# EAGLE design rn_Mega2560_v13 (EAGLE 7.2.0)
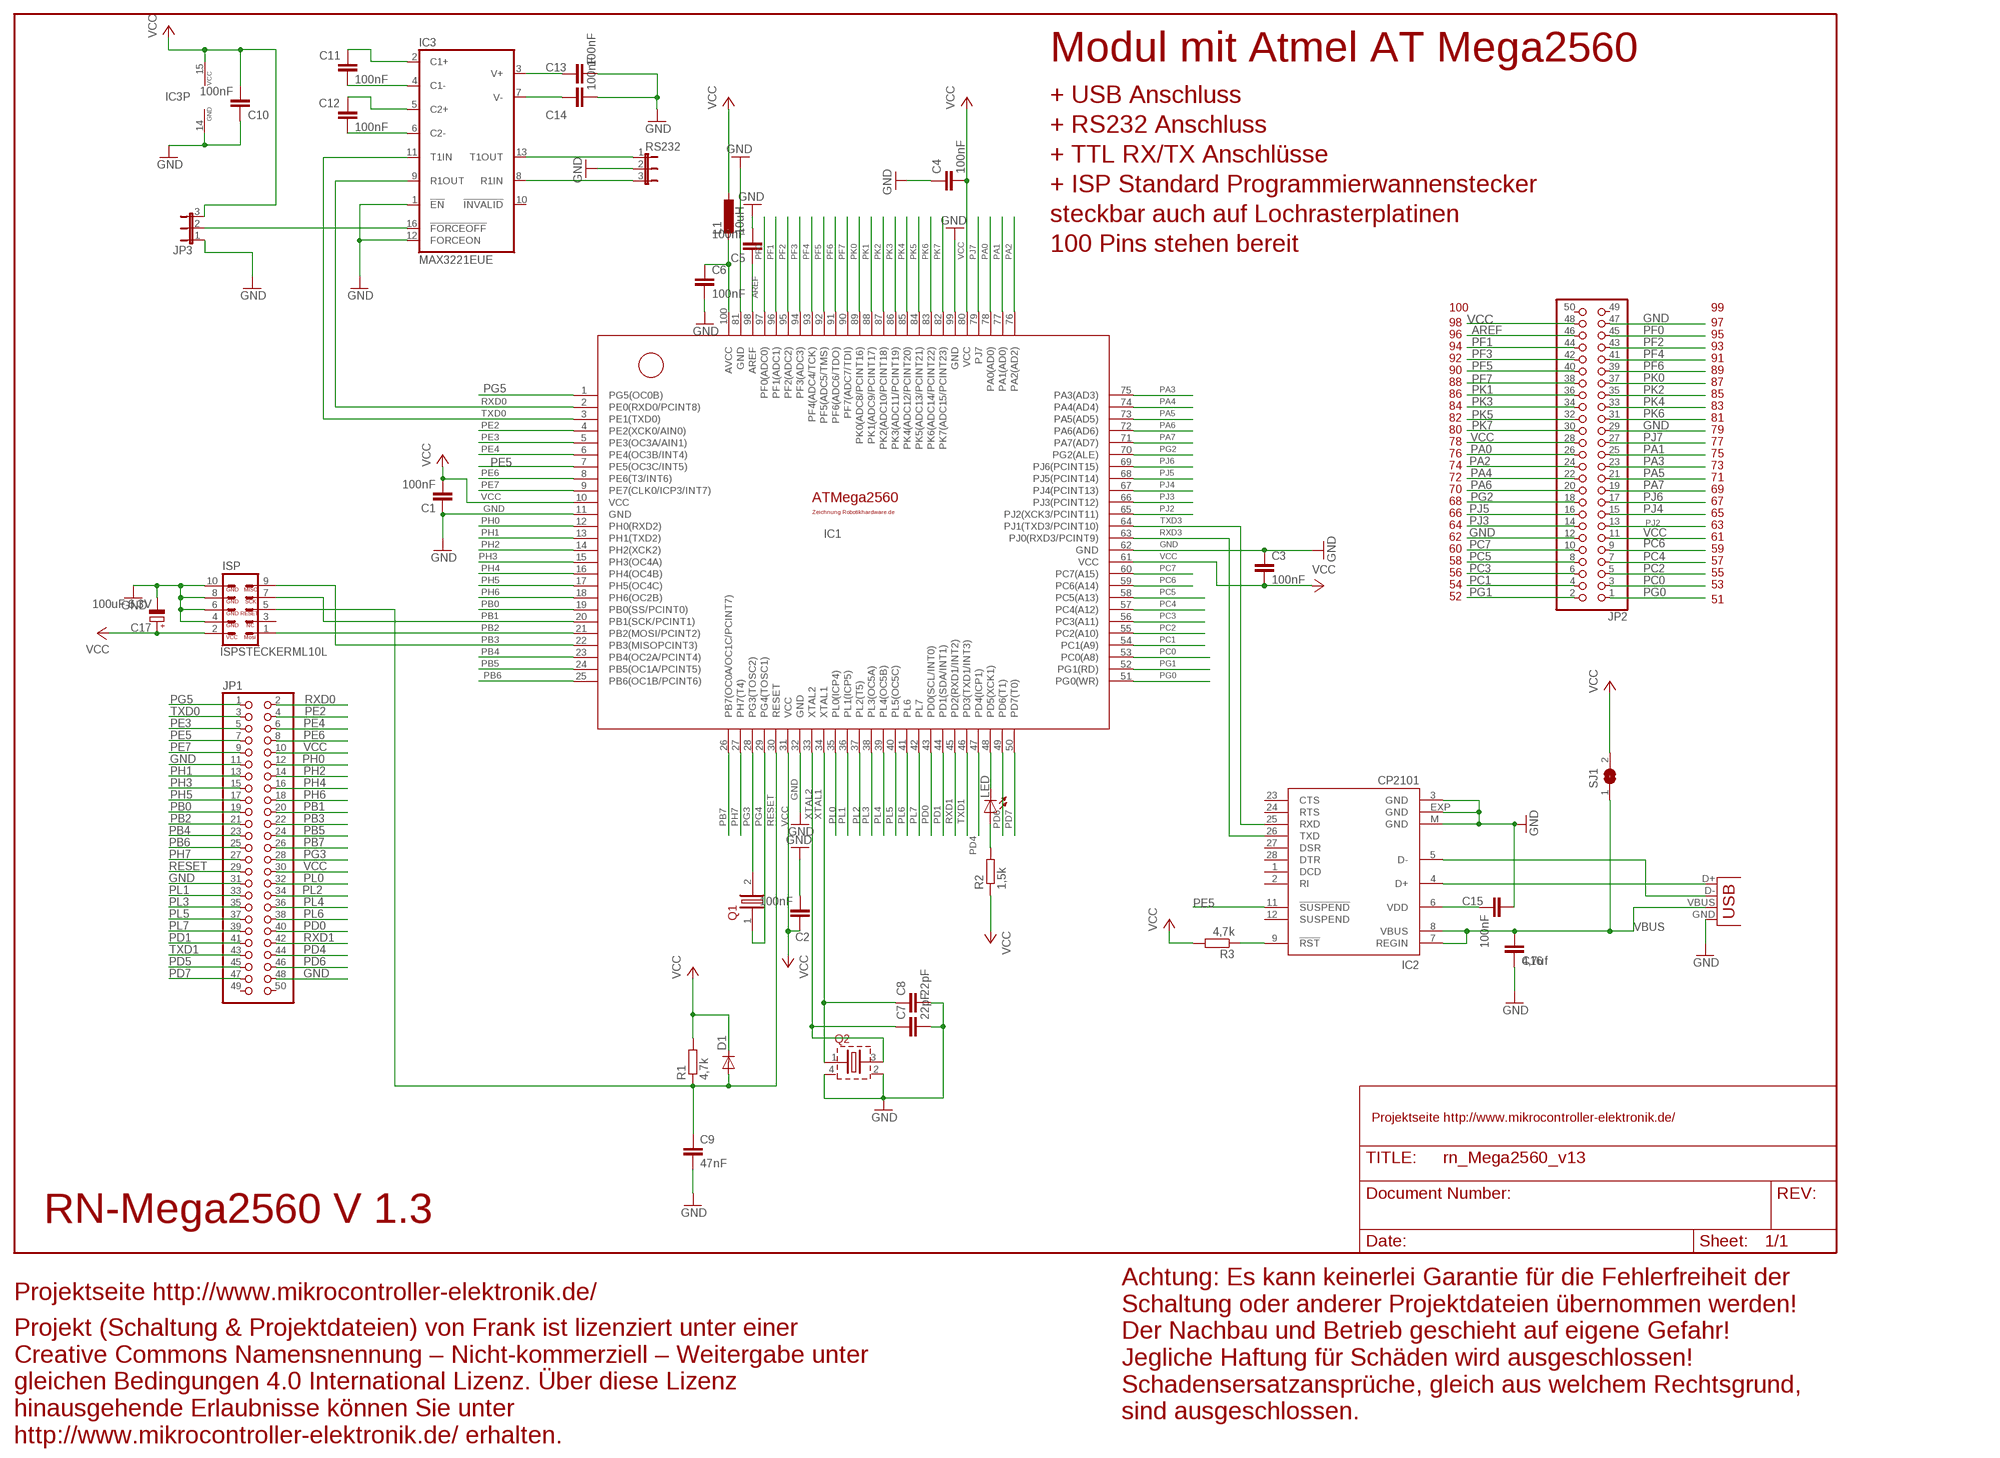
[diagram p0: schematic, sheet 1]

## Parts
C1  100nF  C-EUC0603  [C0603]
C2  100nF  C-EUC0603  [C0603]
C3  100nF  C-EUC0603  [C0603]
C4  100nF  C-EUC0603  [C0603]
C5  100nF  C-EUC0603  [C0603]
C6  100nF  C-EUC0603  [C0603]
C7  22pF  C-EUC0603  [C0603]
C8  22pF  C-EUC0603  [C0603]
C9  47nF  C-EUC0603  [C0603]
C10  100nF  C-EUC0603  [C0603]
C11  100nF  C-EUC0603  [C0603]
C12  100nF  C-EUC0603  [C0603]
C13  100nF  C-EUC0603  [C0603]
C14  100nF  C-EUC0603  [C0603]
C15  100nF  C-EUC0603  [C0603]
C16  4,7uf  C-EUC1206  [C1206]
C17  100uF 6,3V  CPOL-EU085CS-1AR  [085CS_1AR]
D1  DIODE-MINIMELF  [MINIMELF]
IC1  ATMEGA2560PINGLEICH  [TQFP100]
IC2  CP2101  [MLP28]
IC3  MAX3221EUE  [TSSOP16]
ISP  ISPSTECKERML10L  [ML10L]
JP1  PINHD-2X25  [2X25]
JP2  PINHD-2X25  [2X25]
JP3  JP2W  [JP2W]
L1  10uH  L-EUL3225M  [L3225M]
LED  LEDCHIPLED_0805  [CHIPLED_0805]
Q1  FC135QUARZ  [FC135QUARZ]
Q2  KS7QUARZ  [KX7QUARZ]
R1  4,7k  R-EU_M0805  [M0805]
R2  1,5k  R-EU_M0805  [M0805]
R3  4,7k  R-EU_M0805  [M0805]
RS232  JP2W  [JP2W]
SJ1  SJW  [SJW]
USB  USB-MB-H  [USB-MB-H]

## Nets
AREF: C5.1 IC1.98(AREF) JP2.46
AVCC: C6.1 IC1.100(AVCC) L1.2
GND: C1.1 C2.2 C3.1 C4.1 C5.2 C6.2 C7.2 C8.2 C9.2 C10.1 C13.2 C14.2 C15.1 C16.2 C17.- IC1.11(GND) IC1.32(GND) IC1.62(GND) IC1.81(GND) IC1.99(GND) IC2.3(GND) IC2.EXP(GND) IC2.M(GND) IC3.1(!EN) IC3.12(FORCEON) IC3.14(GND) ISP.4 ISP.6 ISP.8 ISP.10 JP1.11 JP1.31 JP1.48 JP2.12 JP2.29 JP2.47 JP3.1 Q2.2(GND) Q2.4(GND) RS232.2 USB.GND
N$9: C12.2 IC3.6(C2-)
N$10: C12.1 IC3.5(C2+)
N$11: C11.2 IC3.4(C1-)
N$12: IC2.5(D-) USB.D-
N$15: C11.1 IC3.2(C1+)
N$16: LED.A R2.2
N$18: IC2.9(!RST) R3.1
N$21: IC3.8(R1IN) RS232.3
N$22: C13.1 IC3.3(V+)
N$23: C14.1 IC3.7(V-)
N$24: IC3.16(!FORCEOFF) JP3.2
N$28: IC2.4(D+) USB.D+
N$29: C15.2 IC2.6(VDD)
PA0: IC1.78(PA0(AD0)) JP2.26
PA1: IC1.77(PA1(AD0)) JP2.25
PA2: IC1.76(PA2(AD2)) JP2.24
PA3: IC1.75(PA3(AD3)) JP2.23
PA4: IC1.74(PA4(AD4)) JP2.22
PA5: IC1.73(PA5(AD5)) JP2.21
PA6: IC1.72(PA6(AD6)) JP2.20
PA7: IC1.71(PA7(AD7)) JP2.19
PB0: IC1.19(PB0(SS/PCINT0)) JP1.19
PB1: IC1.20(PB1(SCK/PCINT1)) ISP.7 JP1.20
PB2: IC1.21(PB2(MOSI/PCINT2)) ISP.1 JP1.21
PB3: IC1.22(PB3(MISOPCINT3)) ISP.9 JP1.22
PB4: IC1.23(PB4(OC2A/PCINT4)) JP1.23
PB5: IC1.24(PB5(OC1A/PCINT5)) JP1.24
PB6: IC1.25(PB6(OC1B/PCINT6)) JP1.25
PB7: IC1.26(PB7(OC0A/OC1C/PCINT7)) JP1.26
PC0: IC1.53(PC0(A8)) JP2.3
PC1: IC1.54(PC1(A9)) JP2.4
PC2: IC1.55(PC2(A10)) JP2.5
PC3: IC1.56(PC3(A11)) JP2.6
PC4: IC1.57(PC4(A12)) JP2.7
PC5: IC1.58(PC5(A13)) JP2.8
PC6: IC1.59(PC6(A14)) JP2.9
PC7: IC1.60(PC7(A15)) JP2.10
PD0: IC1.43(PD0(SCL/INT0)) JP1.40
PD1: IC1.44(PD1(SDA/INT1)) JP1.41
PD4: IC1.47(PD4(ICP1)) JP1.44
PD5: IC1.48(PD5(XCK1)) JP1.45 LED.C
PD6: IC1.49(PD6(T1)) JP1.46
PD7: IC1.50(PD7(T0)) JP1.47
PE2: IC1.4(PE2(XCK0/AIN0)) JP1.4
PE3: IC1.5(PE3(OC3A/AIN1)) JP1.5
PE4: IC1.6(PE4(OC3B/INT4)) JP1.6
PE5: IC1.7(PE5(OC3C/INT5)) IC2.11(!SUSPEND) JP1.7
PE6: IC1.8(PE6(T3/INT6)) JP1.8
PE7: IC1.9(PE7(CLK0/ICP3/INT7)) JP1.9
PF0: IC1.97(PF0(ADC0)) JP2.45
PF1: IC1.96(PF1(ADC1)) JP2.44
PF2: IC1.95(PF2(ADC2)) JP2.43
PF3: IC1.94(PF3(ADC3)) JP2.42
PF4: IC1.93(PF4(ADC4/TCK)) JP2.41
PF5: IC1.92(PF5(ADC5/TMS)) JP2.40
PF6: IC1.91(PF6(ADC6/TDO)) JP2.39
PF7: IC1.90(PF7(ADC7/TDI)) JP2.38
PG0: IC1.51(PG0(WR)) JP2.1
PG1: IC1.52(PG1(RD)) JP2.2
PG2: IC1.70(PG2(ALE)) JP2.18
PG3: IC1.28(PG3(TOSC2)) JP1.28 Q1.2
PG4: IC1.29(PG4(TOSC1)) Q1.1
PG5: IC1.1(PG5(OC0B)) JP1.1
PH0: IC1.12(PH0(RXD2)) JP1.12
PH1: IC1.13(PH1(TXD2)) JP1.13
PH2: IC1.14(PH2(XCK2)) JP1.14
PH3: IC1.15(PH3(OC4A)) JP1.15
PH4: IC1.16(PH4(OC4B)) JP1.16
PH5: IC1.17(PH5(OC4C)) JP1.17
PH6: IC1.18(PH6(OC2B)) JP1.18
PH7: IC1.27(PH7(T4)) JP1.27
PJ2: IC1.65(PJ2(XCK3/PCINT11)) JP2.13
PJ3: IC1.66(PJ3(PCINT12)) JP2.14
PJ4: IC1.67(PJ4(PCINT13)) JP2.15
PJ5: IC1.68(PJ5(PCINT14)) JP2.16
PJ6: IC1.69(PJ6(PCINT15)) JP2.17
PJ7: IC1.79(PJ7) JP2.27
PK0: IC1.89(PK0(ADC8/PCINT16)) JP2.37
PK1: IC1.88(PK1(ADC9/PCINT17)) JP2.36
PK2: IC1.87(PK2(ADC10/PCINT18)) JP2.35
PK3: IC1.86(PK3(ADC11/PCINT19)) JP2.34
PK4: IC1.85(PK4(ADC12/PCINT20)) JP2.33
PK5: IC1.84(PK5(ADC13/PCINT21)) JP2.32
PK6: IC1.83(PK6(ADC14/PCINT22)) JP2.31
PK7: IC1.82(PK7(ADC15/PCINT23)) JP2.30
PL0: IC1.35(PL0(ICP4)) JP1.32
PL1: IC1.36(PL1(ICP5)) JP1.33
PL2: IC1.37(PL2(T5)) JP1.34
PL3: IC1.38(PL3(OC5A)) JP1.35
PL4: IC1.39(PL4(OC5B)) JP1.36
PL5: IC1.40(PL5(OC5C)) JP1.37
PL6: IC1.41(PL6) JP1.38
PL7: IC1.42(PL7) JP1.39
RESET: C9.1 D1.A IC1.30(RESET) ISP.5 JP1.29 R1.1
RXD0: IC1.2(PE0(RXD0/PCINT8)) IC3.9(R1OUT) JP1.2
RXD1: IC1.45(PD2(RXD1/INT2)) JP1.42
RXD3: IC1.63(PJ0(RXD3/PCINT9)) IC2.26(TXD)
T1OUT: IC3.13(T1OUT) RS232.1
TXD0: IC1.3(PE1(TXD0)) IC3.11(T1IN) JP1.3
TXD1: IC1.46(PD3(TXD1/INT3)) JP1.43
TXD3: IC1.64(PJ1(TXD3/PCINT10)) IC2.25(RXD)
VBUS: C16.1 IC2.7(REGIN) IC2.8(VBUS) SJ1.1 USB.VBUS
VCC: C1.2 C2.1 C3.2 C4.2 C10.2 C17.+ D1.C IC1.10(VCC) IC1.31(VCC) IC1.61(VCC) IC1.80(VCC) IC3.15(VCC) ISP.2 JP1.10 JP1.30 JP2.11 JP2.28 JP2.48 JP3.3 L1.1 R1.2 R2.1 R3.2 SJ1.2
XTAL1: C7.1 IC1.33(XTAL2) Q2.3
XTAL2: C8.1 IC1.34(XTAL1) Q2.1
Unconnected: IC2.1(DCD) IC2.2(RI) IC2.12(SUSPEND) IC2.23(CTS) IC2.24(RTS) IC2.27(DSR) IC2.28(DTR) IC3.10(!INVALID) ISP.3 JP1.49 JP1.50 JP2.49 JP2.50

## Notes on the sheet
- Modul mit Atmel AT Mega2560
- + USB Anschluss
- + RS232 Anschluss
- + TTL RX/TX Anschlüsse
- + ISP Standard Programmierwannenstecker
- steckbar auch auf Lochrasterplatinen
- 100 Pins stehen bereit
- 100 | 99
- 98 | 97
- 96 | 95
- 94 | 93
- 92 | 91
- 90 | 89
- 88 | 87
- 86 | 85
- 84 | 83
- 82 | 81
- 80 | 79
- 78 | 77
- 76 | 75
- 74 | 73
- 72 | 71
- 70 | 69
- 68 | 67
- 66 | 65
- 64 | 63
- 62 | 61
- 60 | 59
- 58 | 57
- 56 | 55
- 54 | 53
- 52 | 51
- Projektseite http://www.mikrocontroller-elektronik.de/
- RN-Mega2560 V 1.3
- Projektseite http://www.mikrocontroller-elektronik.de/
- Achtung: Es kann keinerlei Garantie für die Fehlerfreiheit der
  Schaltung oder anderer Projektdateien übernommen werden!
  Der Nachbau und Betrieb geschieht auf eigene Gefahr! 
  Jegliche Haftung für Schäden wird ausgeschlossen!
  Schadensersatzansprüche, gleich aus welchem Rechtsgrund,
  sind ausgeschlossen.
- Projekt (Schaltung & Projektdateien) von Frank ist lizenziert unter einer
  Creative Commons Namensnennung – Nicht-kommerziell – Weitergabe unter
  gleichen Bedingungen 4.0 International Lizenz. Über diese Lizenz
  hinausgehende Erlaubnisse können Sie unter
  http://www.mikrocontroller-elektronik.de/ erhalten.

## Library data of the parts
C1-C16 = rcl:C-EU: CAPACITOR, European symbol
C17 = rcl:CPOL-EU: POLARIZED CAPACITOR, European symbol
D1 = diode:DIODE-: DIODE
IC1 = RoboterNetz:ATMEGA2560PINGLEICH
IC2 = silabs:CP210*: Single-Chip USB to UART Bridge Source: www.silabs.com .. CP2101.pdf / cp2102.pdf
IC3 = maxim:MAX3221*: RS-232 Transceivers with AutoShutdown 1µA Supply-Current, True +3V to +5.5V http://dbserv.maxim-ic.com/
ISP = RoboterNetz:ISPSTECKER
JP1 JP2 = pinhead:PINHD-2X25: PIN HEADER
JP3 RS232 = jumper:JP2W: JUMPER
L1 = rcl:L-EU: INDUCTOR, European symbol
LED = led:LED: LED
Q1 = RoboterNetz:FC135QUARZ
Q2 = RoboterNetz:KS7QUARZ
R1-R3 = rcl:R-EU_: RESISTOR, European symbol
SJ1 = jumper:SJ: SMD solder JUMPER
USB = con-usb:USB: USB Connectors

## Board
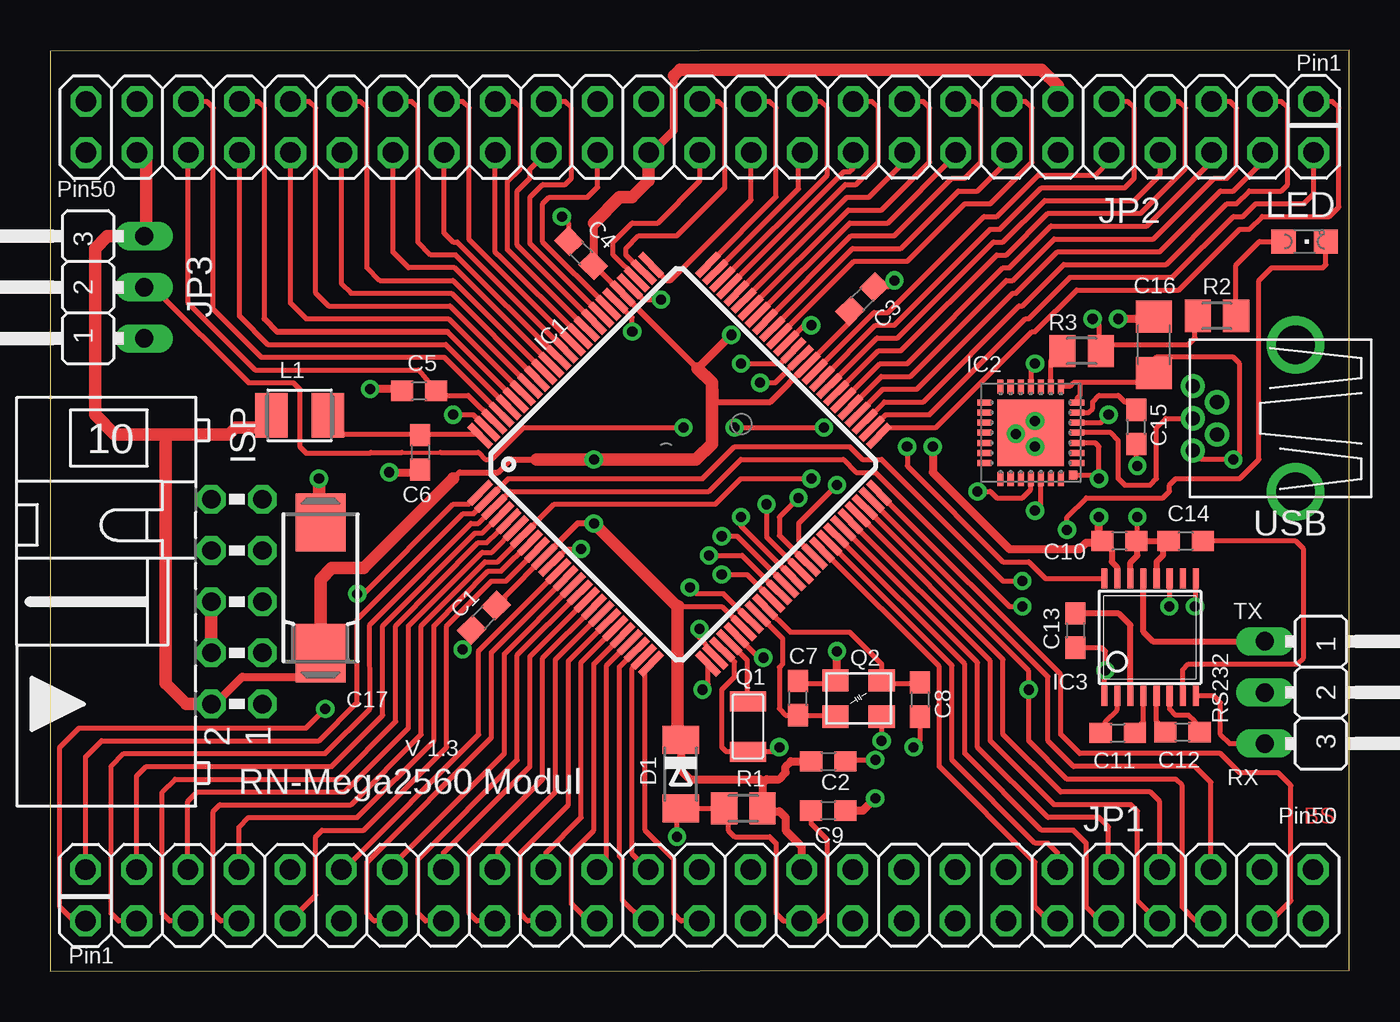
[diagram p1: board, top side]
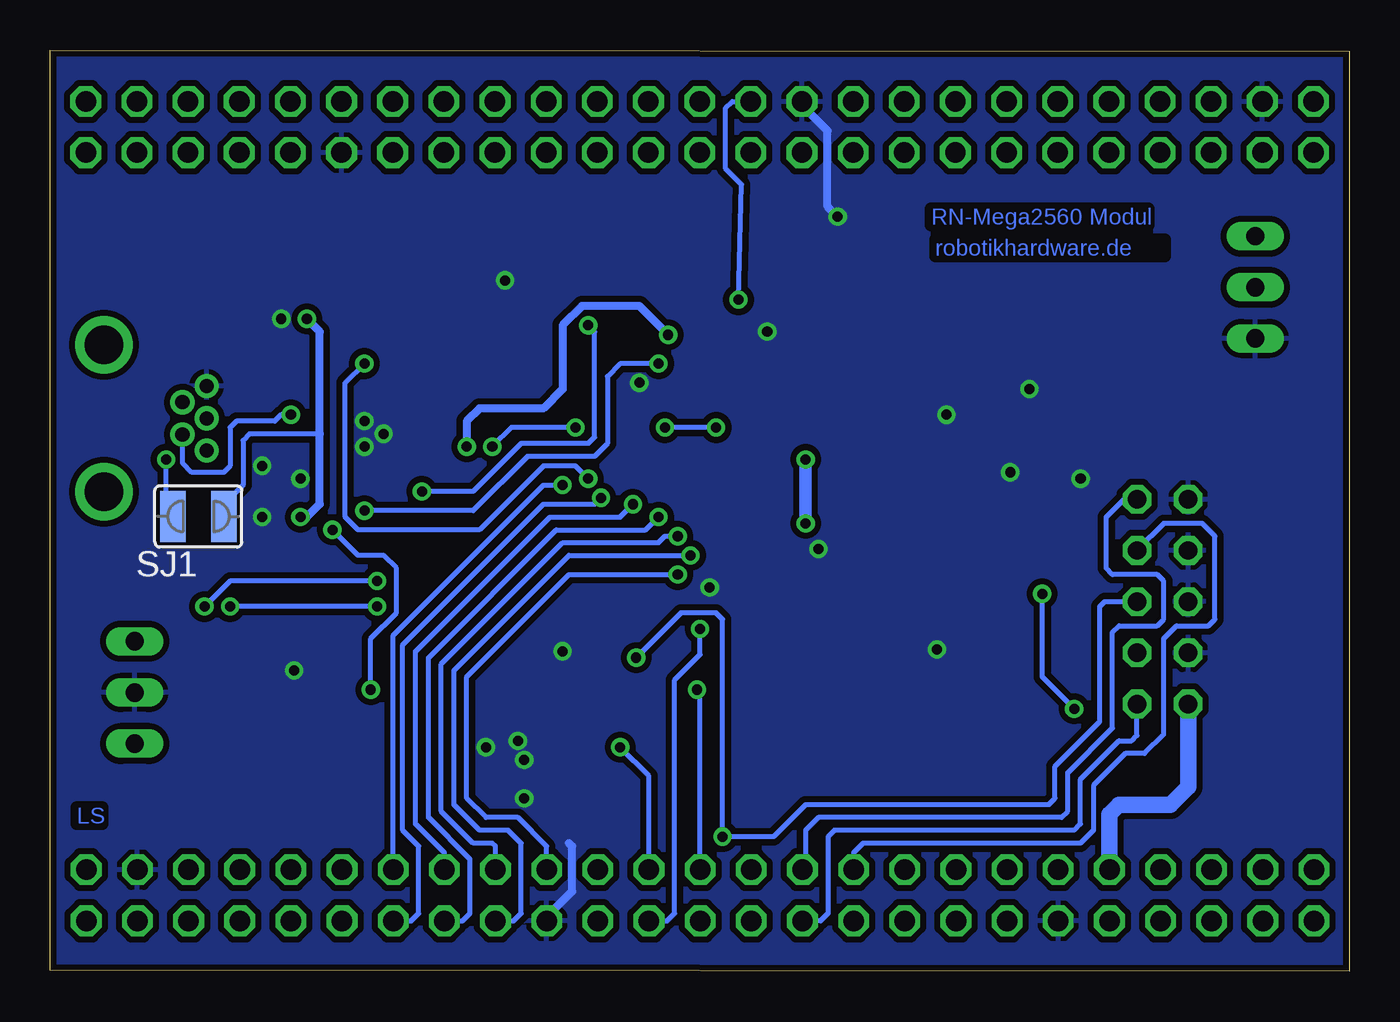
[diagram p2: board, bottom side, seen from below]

Size 64.49 x 45.73 mm. Coordinates in mm from the lower left corner, seen from the top.
Outline: 0,0 64.49,0.04 64.49,45.73 0,45.69 0,0
Copper layers (1*16): Top 0.035mm / dielectric 1.5mm / Bottom 0.035mm
Design rules "minimegaboard": minimum track width 8mil, minimum drill 10mil, track to track 6mil, track to pad 4mil, pad to pad 4mil, via to via 8mil, smd to smd 8mil, copper to edge 10mil, drill to drill 8mil, minimum pad ring 10mil, minimum via ring 8mil, stop-mask expansion 4mil, vias tented up to drill 0mil, thermal gap 10mil
bRestrict: area 55.2,21.3 to 59.1,23.8

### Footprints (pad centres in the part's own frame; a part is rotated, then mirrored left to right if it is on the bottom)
C0603 = smd 1.1 x 1: 1 -0.85,0; 2 0.85,0
C1206 = smd 1.6 x 1.8: 1 -1.4,0; 2 1.4,0
085CS_1AR = smd 2.9 x 2.5: + 3.25,0; - -3.25,0
MINIMELF = smd 1.4 x 1.8: A 1.7,0; C -1.7,0
TQFP100 = smd 1.5 x 0.35: 1 -8,6; 2 -8,5.5; 3 -8,5; 4 -8,4.5; 5 -8,4; 6 -8,3.5; 7 -8,3; 8 -8,2.5; 9 -8,2; 10 -8,1.5; 11 -8,1; 12 -8,0.5; 13 -8,0; 14 -8,-0.5; 15 -8,-1; 16 -8,-1.5; 17 -8,-2; 18 -8,-2.5; 19 -8,-3; 20 -8,-3.5; 21 -8,-4; 22 -8,-4.5; 23 -8,-5; 24 -8,-5.5; 25 -8,-6; 51 8,-6; 52 8,-5.5; 53 8,-5; 54 8,-4.5; 55 8,-4; 56 8,-3.5; 57 8,-3; 58 8,-2.5; 59 8,-2; 60 8,-1.5; 61 8,-1; 62 8,-0.5; 63 8,0; 64 8,0.5; 65 8,1; 66 8,1.5; 67 8,2; 68 8,2.5; 69 8,3; 70 8,3.5; 71 8,4; 72 8,4.5; 73 8,5; 74 8,5.5; 75 8,6 | smd 0.35 x 1.5: 26 -6,-8; 27 -5.5,-8; 28 -5,-8; 29 -4.5,-8; 30 -4,-8; 31 -3.5,-8; 32 -3,-8; 33 -2.5,-8; 34 -2,-8; 35 -1.5,-8; 36 -1,-8; 37 -0.5,-8; 38 0,-8; 39 0.5,-8; 40 1,-8; 41 1.5,-8; 42 2,-8; 43 2.5,-8; 44 3,-8; 45 3.5,-8; 46 4,-8; 47 4.5,-8; 48 5,-8; 49 5.5,-8; 50 6,-8; 76 6,8; 77 5.5,8; 78 5,8; 79 4.5,8; 80 4,8; 81 3.5,8; 82 3,8; 83 2.5,8; 84 2,8; 85 1.5,8; 86 1,8; 87 0.5,8; 88 0,8; 89 -0.5,8; 90 -1,8; 91 -1.5,8; 92 -2,8; 93 -2.5,8; 94 -3,8; 95 -3.5,8; 96 -4,8; 97 -4.5,8; 98 -5,8; 99 -5.5,8; 100 -6,8
MLP28 = smd 0.7 x 0.3: 1 -2.3,1.5; 2 -2.3,1; 3 -2.3,0.5; 4 -2.3,0; 5 -2.3,-0.5; 6 -2.3,-1; 7 -2.3,-1.5; 15 2.3,-1.5; 16 2.3,-1; 17 2.3,-0.5; 18 2.3,0; 19 2.3,0.5; 20 2.3,1; 21 2.3,1.5 | smd 0.3 x 0.7: 8 -1.5,-2.3; 9 -1,-2.3; 10 -0.5,-2.3; 11 0,-2.3; 12 0.5,-2.3; 13 1,-2.3; 14 1.5,-2.3; 22 1.5,2.3; 23 1,2.3; 24 0.5,2.3; 25 0,2.3; 26 -0.5,2.3; 27 -1,2.3; 28 -1.5,2.3 | smd 3.3 x 3.3: EXP 0,0 | smd 0.435 x 0.435: M -2.103,2.103
TSSOP16 = smd 0.305 x 0.991: 1 -2.275,-2.918; 2 -1.625,-2.918; 3 -0.975,-2.918; 4 -0.325,-2.918; 5 0.325,-2.918; 6 0.975,-2.918; 7 1.625,-2.918; 8 2.275,-2.918; 9 2.275,2.918; 10 1.625,2.918; 11 0.975,2.918; 12 0.325,2.918; 13 -0.325,2.918; 14 -0.975,2.918; 15 -1.625,2.918; 16 -2.275,2.918
ML10L = drill 0.914 octagon: 1 -5.08,-1.27; 2 -5.08,1.27; 3 -2.54,-1.27; 4 -2.54,1.27; 5 0,-1.27; 6 0,1.27; 7 2.54,-1.27; 8 2.54,1.27; 9 5.08,-1.27; 10 5.08,1.27
2X25 = drill 1.016 octagon: 1 -30.48,-1.27; 2 -30.48,1.27; 3 -27.94,-1.27; 4 -27.94,1.27; 5 -25.4,-1.27; 6 -25.4,1.27; 7 -22.86,-1.27; 8 -22.86,1.27; 9 -20.32,-1.27; 10 -20.32,1.27; 11 -17.78,-1.27; 12 -17.78,1.27; 13 -15.24,-1.27; 14 -15.24,1.27; 15 -12.7,-1.27; 16 -12.7,1.27; 17 -10.16,-1.27; 18 -10.16,1.27; 19 -7.62,-1.27; 20 -7.62,1.27; 21 -5.08,-1.27; 22 -5.08,1.27; 23 -2.54,-1.27; 24 -2.54,1.27; 25 0,-1.27; 26 0,1.27; 27 2.54,-1.27; 28 2.54,1.27; 29 5.08,-1.27; 30 5.08,1.27; 31 7.62,-1.27; 32 7.62,1.27; 33 10.16,-1.27; 34 10.16,1.27; 35 12.7,-1.27; 36 12.7,1.27; 37 15.24,-1.27; 38 15.24,1.27; 39 17.78,-1.27; 40 17.78,1.27; 41 20.32,-1.27; 42 20.32,1.27; 43 22.86,-1.27; 44 22.86,1.27; 45 25.4,-1.27; 46 25.4,1.27; 47 27.94,-1.27; 48 27.94,1.27; 49 30.48,-1.27; 50 30.48,1.27
JP2W = drill 0.914 long: 1 -2.54,-1.27; 2 0,-1.27; 3 2.54,-1.27
L3225M = smd 1.6 x 2.2: 1 -1.4,0; 2 1.4,0
CHIPLED_0805 = smd 1.2 x 1.2: A 0,-1.05; C 0,1.05
FC135QUARZ = smd 1 x 1.8: 1 -2.3,-0.2; 2 0.2,-0.2
KX7QUARZ = smd 1.3 x 1.1: 1 -1.09,-0.8; 2 1.21,-0.8; 3 1.21,1; 4 -1.09,1
M0805 = smd 1.3 x 1.6: 1 -0.95,0; 2 0.95,0
SJW = smd 1.27 x 2.54: 1 -1.27,0; 2 1.27,0
USB-MB-H = drill 0.7 pad 1.2: D+ 5.1,0; D- 3.9,0.8; GND 5.1,-1.6; ID 3.9,-0.8; VBUS 5.1,1.6 | drill 1.9: P$6 0,-3.65; P$7 0,3.65

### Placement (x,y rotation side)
C1  21.52,17.56 45 top
C2  38.63,10.42 0 top
C3  40.31,33.39 225 top
C4  26.36,35.65 315 top
C5  18.31,28.82 180 top
C6  18.36,25.77 270 top
C7  37.13,13.56 90 top
C8  43.18,13.49 270 top
C9  38.62,7.98 0 top
C10  53.08,21.37 180 top
C11  52.99,11.83 0 top
C12  56.21,11.87 0 top
C13  50.89,16.92 270 top
C14  56.37,21.36 180 top
C15  53.93,27.03 90 top
C16  54.79,31.11 90 top
C17  13.42,19.04 270 top
D1  31.31,9.79 270 top
IC1  31.24,25.17 45 top
IC2  48.68,26.74 180 top
IC3  54.6,16.58 0 top
ISP  9.26,18.35 90 top
JP1  32.22,3.77 0 top
JP2  32.25,41.92 180 top
JP3  3.39,33.96 90 top
L1  12.38,27.6 0 top
LED  62.28,36.24 270 top
Q1  34.84,11.1 270 top
Q2  40.19,13.65 180 top
R1  34.41,8.09 0 top
R2  57.92,32.54 0 top
R3  51.2,30.8 0 top
RS232  61.57,13.84 270 top
SJ1  57.14,22.59 0 bottom
USB  61.83,27.46 180 top

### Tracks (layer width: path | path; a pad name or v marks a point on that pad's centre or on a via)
AREF
  Top 0.254: JP2.46 6.85,33.17 10.16,29.86 18.28,29.86 C5.1 19.37,28.55 19.37,28.59 20.75,28.59 IC1.98
AVCC
  Top 0.254: L1.2 13.78,26.68 18.3,26.68 C6.1 18.41,26.68 21.25,26.68 IC1.100
GND  (via drill 0.5)
  Top 0.254: IC2.M 51.93,24.64 v52.07,24.46 52.07,26.05 51.88,26.24 IC2.3 | C4.1 25.75,37.12 v25.4,37.48 | IC1.81 28.89,32.47 v28.89,31.76 | IC1.62 36,29.22 v35.24,29.22 | C3.1 41.59,33.99 v41.91,34.3 | IC1.11 25.62,20.97 v26.35,20.97 | C6.2 18.41,24.87 | C10.1 53.98,21.29 v53.98,22.56 | Q2.2 38.83,14.3 37.15,14.3 37.15,14.39 C7.2 37.15,14.43 | C2.2 39.44,10.42 39.37,10.49 v40.96,10.49 | Q2.4 41.28,12.71 41.27,12.71 v41.27,11.44 | C8.2 43.18,11.45 v42.86,11.13 | 50.8,16.07 C13.2 52.21,16.07 52.39,15.89 v52.39,14.93 52.33,14.87 IC3.1 | IC1.99 21,27.63 v20,27.63 | IC1.32 33.42,18.75 32.07,18.75 v31.75,19.06 | C1.1 20.95,16.92 20.95,16.46 v20.47,15.98 | IC2.EXP 48.68,26.26 v48.9,26.05 | C15.1 53.93,25.14 v53.98,25.09
  Top 0.305: IC3.14 53.63,20.3 53.98,20.65 53.98,21.29 53.93,21.33 C10.1 55.48,21.37 55.56,21.29 | IC3.12 54.92,20.33 55.24,20.65 55.24,20.97 55.56,21.29 | 55.56,21.29 55.52,21.32 C14.2
  Top 0.406: C9.2 40.35,7.98 v40.96,8.58 | Q2.2 38.98,14.54 39.05,14.62 v39.05,15.89 | C6.2 18.24,24.92 18.1,24.78 v16.83,24.78 | C5.2 17.55,28.82 17.46,28.9 v15.88,28.9 | C16.2 54.72,32.82 54.29,32.4 v53.02,32.4
  Top 0.61: C17.- 13.42,22.47 13.34,22.56 v13.34,24.46 | 7.99,18.38 ISP.6 | ISP.4 7.99,18.38 | 7.99,18.38 7.94,18.43
  Bottom 0.406: JP2.29 27.17,43.01 25.89,41.73 25.89,37.97 v25.4,37.48 | JP1.31 39.84,2.7 38.58,3.96 38.58,6.21 38.73,6.36
  other vias: 47.94,26.68 48.9,27.32
  pour Bottom (isolate 0.305): 0,0.01 0,45.42 19.05,45.42 64.14,45.42 64.14,0.33 0,0.33
N$9
  Top 0.254: IC3.6 55.58,13.02 55.88,12.71 56.52,12.71 56.83,12.4 56.83,12.08 57.06,11.85 | 57.06,11.85 57.15,11.76 | C12.2 57.06,11.85
N$10
  Top 0.254: C12.1 55.36,11.96 54.92,12.4 IC3.5
N$11
  Top 0.254: C11.2 53.84,11.95 54.28,12.38 IC3.4
N$12  (via drill 0.5)
  Top 0.254: IC2.5 52.15,27.24 v52.55,27.63
  Bottom 0.254: v52.55,27.63 53.02,27.63 53.34,27.32 55.24,27.32 55.56,27 55.56,25.09 55.88,24.78 57.47,24.78 57.93,25.24 USB.D-
N$15
  Top 0.254: IC3.2 52.98,12.98 52.39,12.4 52.39,12.08 C11.1 | C11.1 52.07,11.76 | C11.1
N$16
  Top 0.254: R2.2 58.87,35.07 60.04,36.24 LED.A
N$18
  Top 0.254: R3.1 50.18,30.8 50.16,30.81 49.68,30.32 IC2.9
N$21
  Top 0.254: IC3.8 57.79,13.66 58.1,13.35 58.1,11.76 58.56,11.3 RS232.3
N$22
  Top 0.305: C13.1 53.05,17.77 53.63,17.19 IC3.3
N$23
  Top 0.254: IC3.7 56.23,14.96 56.52,15.25 61.91,15.25 62.23,15.57 62.23,20.97 61.84,21.36 C14.1
N$24  (via drill 0.5)
  Top 0.2: 17.46,25.77 19.37,25.77
  Top 0.254: IC3.16 49.41,19.5 48.58,20.33 47.31,20.33 42.55,25.09 v42.55,26.05 | JP3.2 4.74,33.96 5.08,33.98 9.84,29.22 12.06,29.22 12.38,28.9 12.38,26.05 12.7,25.73 15.88,25.73 15.91,25.77 17.46,25.77 | v33.97,27 v38.42,27 | v31.43,27 23.5,27 21.91,25.41 21.59,25.41 21.25,25.77 19.37,25.77
  Bottom 0.254: v42.55,26.05 41.59,27 v38.42,27 | v31.43,27 v33.97,27
N$28
  Top 0.254: IC2.4 52.65,26.74 53.02,26.36 53.02,24.46 53.34,24.14 54.61,24.14 54.93,24.46 54.93,27 55.38,27.45 USB.D+
N$29
  Top 0.254: IC2.6 51.54,27.74 51.75,27.95 51.75,28.27 52.07,28.59 53.02,28.59 53.34,28.27 53.66,28.27 53.93,28 C15.2
PA0
  Top 0.254: JP2.26 32.25,39.25 30.16,37.16 28.89,37.16 27.94,36.21 27.94,35.57 29.12,34.39 IC1.78
PA1
  Top 0.254: IC1.77 29.43,34.72 28.57,35.57 28.57,35.89 29.21,36.53 31.11,36.53 33.5,38.91 33.5,42.87 33.18,43.19 JP2.25
PA2
  Top 0.254: IC1.76 30.59,34.3 30.8,34.3 34.79,38.29 JP2.24
PA3
  Top 0.254: IC1.75 36.04,38.45 36.04,42.87 35.72,43.19 JP2.23
PA4
  Top 0.254: IC1.74 37.15,38.86 37.15,40.47 JP2.22
PA5
  Top 0.254: IC1.73 33.4,34.36 38.58,39.54 38.58,42.87 38.26,43.19 JP2.21
PA6
  Top 0.254: IC1.72 39.4,39.7 39.69,39.7 39.87,39.88 JP2.20
PA7
  Top 0.254: IC1.71 39.48,39.07 40.01,39.07 41.12,40.18 41.12,42.87 40.8,43.19 JP2.19
PB0
  Top 0.254: IC1.19 25.72,15.41 25.72,8.27 23.34,5.89 23.34,2.87 23.7,2.5 JP1.19
PB1
  Top 0.254: IC1.20 26.35,15.34 26.35,7.63 24.61,5.88 JP1.20
  Bottom 0.254: JP1.20 24.61,5.89 24.13,6.36 13.34,6.36 12.7,7 12.7,9.22 11.11,10.81 10.16,10.81 9.21,11.76 9.21,16.52 8.57,17.16 6.99,17.16 6.67,17.47 6.67,21.6 7.3,22.24 9.21,22.24 10.53,20.91 ISP.7
PB2
  Top 0.254: IC1.21 26.99,15.26 26.99,7 25.88,5.89 25.88,3.35 26.56,2.66 JP1.21
  Bottom 0.254: ISP.1 10.53,11.71 10.79,11.44 11.43,11.44 13.34,9.54 13.34,7.32 13.65,7 25.56,7 25.88,6.68 25.88,2.87 26.25,2.5 JP1.21
PB3
  Top 0.254: IC1.22 27.62,15.19 27.62,5.52 JP1.22
  Bottom 0.254: ISP.9 11.19,23.43 12.06,22.56 12.06,20.02 11.75,19.7 9.53,19.7 9.21,19.38 9.21,17.47 9.53,17.16 11.43,17.16 11.75,16.84 11.75,12.08 13.97,9.85 13.97,7.95 14.29,7.63 26.35,7.63 26.99,7 26.99,5.73 27.14,5.57 JP1.22
PB4
  Top 0.254: JP1.23 29.42,2.5 28.42,3.51 28.42,5.57 28.26,5.73 28.26,15.12 IC1.23
PB5
  Top 0.254: IC1.24 28.89,15.05 28.89,5.83 JP1.24
PB6
  Top 0.254: IC1.25 29.53,14.97 29.53,7 30.96,5.57 30.96,2.87 31.32,2.5 JP1.25
PB7  (via drill 0.5)
  Top 0.254: IC1.26 32.65,14.25 v32.38,13.98
  Bottom 0.254: JP1.26 32.23,13.82 v32.38,13.98
PC0
  Top 0.254: JP2.3 61.12,43.19 61.44,42.87 61.44,39.07 61.12,38.75 59.53,38.75 58.9,38.11 58.42,38.11 58.1,37.79 55.4,35.1 50.32,35.1 48.26,33.03 48.1,33.03 43.34,28.27 41.41,28.27 IC1.53
PC1
  Top 0.254: IC1.54 41.34,28.9 43.02,28.9 47.78,33.67 47.94,33.67 50.01,35.73 55.09,35.73 58.1,38.75 58.74,38.75 60.19,40.2 JP2.4
PC2
  Top 0.254: IC1.55 41.26,29.54 42.7,29.54 47.47,34.3 47.78,34.3 49.85,36.37 54.77,36.37 57.78,39.38 58.42,39.38 58.9,39.86 58.9,42.87 58.58,43.19 JP2.5
PC3
  Top 0.254: IC1.56 41.19,30.18 42.55,30.18 47.31,34.94 47.62,34.94 49.69,37 54.45,37 57.65,40.2 JP2.6
PC4
  Top 0.254: JP2.7 56.04,43.19 56.36,42.87 56.36,39.86 54.13,37.64 49.53,37.64 47.47,35.57 46.99,35.57 42.23,30.81 41.12,30.81 IC1.57
PC5
  Top 0.254: JP2.8 55.11,39.57 53.82,38.27 49.37,38.27 47.31,36.21 46.83,36.21 42.07,31.45 41.05,31.45 IC1.58
PC6
  Top 0.254: JP2.9 53.5,43.19 53.82,42.87 53.82,39.38 53.34,38.91 49.21,38.91 47.15,36.84 46.67,36.84 41.91,32.08 40.98,32.08 IC1.59
PC7
  Top 0.254: JP2.10 52.57,40.2 51.91,39.54 49.05,39.54 46.99,37.48 46.35,37.48 41.59,32.72 40.9,32.72 IC1.60
PD0
  Top 0.254: IC1.43 44.77,15.18 44.77,10.49 48.9,6.36 49.53,6.36 50.01,5.89 JP1.40
PD1
  Top 0.254: IC1.44 45.4,15.25 45.4,10.81 49.21,7 50.8,7 51.44,6.36 51.44,3.19 52.12,2.5 JP1.41
PD4
  Top 0.254: IC1.47 40.09,22.7 47.31,15.48 47.31,11.76 50.16,8.9 54.61,8.9 55.09,8.43 JP1.44
PD5  (via drill 0.5)
  Top 0.254: IC1.48 48.58,14.91 v48.58,13.98 48.58,11.44 50.48,9.54 55.88,9.54 56.2,9.22 56.2,3.19 56.88,2.5 JP1.45 | LED.C 63.33,35.08 63.18,34.94 60.64,34.94 60.01,34.3 60.01,25.41 59.05,24.46 55.88,24.46 55.56,24.14 55.56,23.82 55.24,23.51 51.44,23.51 50.48,22.56 v50.48,21.92
  Bottom 0.254: v50.48,21.92 49.21,20.65 47.94,20.65 47.31,20.02 47.31,17.79 48.58,16.52 v48.58,13.98
PD6
  Top 0.254: IC1.49 40.79,23.36 49.53,14.62 49.53,11.44 50.8,10.17 56.83,10.17 57.62,9.38 JP1.46
PD7
  Top 0.254: IC1.50 50.16,14.73 50.16,11.76 51.12,10.81 58.1,10.81 59.05,9.85 60.96,9.85 61.59,9.22 61.59,3.51 60.59,2.5 JP1.47
PE2
  Top 0.254: JP1.4 4.29,9.69 4.76,10.17 13.97,10.17 16.51,12.71 16.51,17.16 21.08,21.75 21.43,21.75 IC1.4
PE3
  Top 0.254: JP1.5 5.92,2.5 5.56,2.87 5.56,8.9 6.19,9.54 14.29,9.54 17.14,12.4 17.14,17.16 21.25,21.29 21.67,21.29 IC1.5
PE4
  Top 0.254: IC1.6 21.93,20.8 21.44,20.8 17.78,17.16 17.78,12.08 14.61,8.9 7.3,8.9 6.83,8.42 JP1.6
PE5  (via drill 0.5)
  Top 0.254: JP1.7 8.46,2.5 8.1,2.87 8.1,7.95 8.41,8.27 14.92,8.27 18.41,11.76 18.41,17.16 21.58,20.33 22.21,20.33 23.18,21.29 23.18,21.35 IC1.7 25.02,23.19 33.02,23.19 34.29,24.46 v37.78,24.46 | IC2.11 48.68,29.96 v48.9,30.18
  Bottom 0.254: v37.78,24.46 38.42,25.09 40.01,25.09 43.18,21.92 49.21,21.92 49.85,22.56 49.85,29.22 v48.9,30.18
PE6
  Top 0.254: IC1.8 22.38,19.88 21.74,19.88 19.05,17.16 19.05,11.44 15.24,7.63 9.84,7.63 9.37,7.15 JP1.8
PE7
  Top 0.254: JP1.9 13.18,3.77 13.18,6.68 13.49,7 15.56,7 19.68,11.13 19.68,17.16 21.91,19.38 22.62,19.38 IC1.9
PF0
  Top 0.254: JP2.45 7.78,43.19 8.1,42.87 8.1,32.87 10.48,30.49 19.56,30.49 IC1.97
PF1
  Top 0.254: IC1.96 19.63,31.13 10.79,31.13 9.39,32.53 JP2.44
PF2
  Top 0.254: 19.7,31.76 IC1.95 | JP2.43 10.32,43.19 10.64,42.87 10.64,32.4
  Top 0.305: 19.7,31.76 11.27,31.76 10.64,32.4
PF3
  Top 0.254: IC1.94 19.77,32.4 12.7,32.4 11.93,33.17 JP2.42
PF4
  Top 0.254: IC1.93 19.84,33.03 13.81,33.03 13.18,33.67 13.18,42.87 12.86,43.19 JP2.41
PF5
  Top 0.254: IC1.92 19.92,33.67 14.92,33.67 14.47,34.12 JP2.40
PF6
  Top 0.254: IC1.91 19.99,34.3 16.35,34.3 15.72,34.94 15.72,42.87 15.4,43.19 JP2.39
PF7
  Top 0.254: IC1.90 20.06,34.94 17.78,34.94 17.01,35.71 JP2.38
PG0
  Top 0.254: JP2.1 63.66,43.19 63.98,42.87 63.98,37.95 63.5,37.48 60.17,37.48 59.53,36.84 59.05,36.84 56.04,33.83 50.96,33.83 48.9,31.76 48.74,31.76 43.97,27 41.55,27 IC1.51
PG1
  Top 0.254: IC1.52 41.48,27.63 43.66,27.63 48.42,32.4 48.58,32.4 50.64,34.46 55.72,34.46 58.74,37.48 59.21,37.48 59.85,38.11 62.23,38.11 62.73,38.61 JP2.2
PG2
  Top 0.254: IC1.70 39.55,38.43 40.64,38.43 42.41,40.2 JP2.18
PG3  (via drill 0.5)
  Top 0.254: IC1.28 33.97,15.37 33.97,14.62 33.34,13.98 33.34,11.13 33.56,10.9 Q1.2 35.97,10.9 v36.2,11.13
  Bottom 0.254: JP1.28 34.77,9.69 v36.2,11.13
PG4
  Top 0.254: 34.61,13.05 34.61,13.35 | Q1.1 34.61,13.05 | IC1.29 34.61,15.44 34.61,13.05
PG5  (via drill 0.5)
  Top 0.254: JP1.1 1.16,2.5 0.48,3.19 0.48,11.13 1.43,12.08 12.7,12.08 v13.65,13.03 | IC1.1 20.77,23.19 20,23.19 15.56,18.75 v15.24,18.75
  Bottom 0.254: v13.65,13.03 15.24,14.62 v15.24,18.75
PH0
  Top 0.254: IC1.12 21.27,15.91 21.27,11.76 14.55,5.04 JP1.12
PH1
  Top 0.254: IC1.13 21.91,15.84 21.91,11.6 15.72,5.41 15.72,2.87 16.08,2.5 JP1.13
PH2
  Top 0.254: IC1.14 22.54,15.77 22.54,10.81 16.98,5.25 JP1.14
PH3
  Top 0.254: IC1.15 23.18,15.7 23.18,10.49 18.26,5.57 18.26,2.87 18.62,2.5 JP1.15
PH4
  Top 0.254: IC1.16 23.81,15.62 23.81,10.17 19.52,5.88 JP1.16
PH5
  Top 0.254: IC1.17 24.45,15.55 24.45,9.54 20.8,5.89 20.8,2.87 21.16,2.5 JP1.17
PH6
  Top 0.254: IC1.18 25.08,15.48 25.08,8.9 22.23,6.04 22.23,5.2 JP1.18
PH7  (via drill 0.5)
  Top 0.254: IC1.27 32.23,16.57 v32.23,17
  Bottom 0.254: v32.23,17 32.23,15.73 33.5,14.46 33.5,2.87 33.86,2.5 JP1.27
PJ2
  Top 0.254: IC1.65 39.91,35.25 42.55,35.25 45.4,38.11 46.67,38.11 48.74,40.18 48.74,42.87 48.42,43.19 JP2.13
PJ3
  Top 0.254: IC1.66 39.84,35.89 42.23,35.89 45.09,38.75 46.04,38.75 47.49,40.2 JP2.14
PJ4
  Top 0.254: IC1.67 39.76,36.53 41.91,36.53 44.77,39.38 45.4,39.38 46.2,40.18 46.2,42.87 45.88,43.19 JP2.15
PJ5
  Top 0.254: IC1.68 39.69,37.16 41.59,37.16 44.95,40.52 JP2.16
PJ6
  Top 0.254: IC1.69 39.62,37.79 41.27,37.79 43.66,40.18 43.66,42.87 43.34,43.19 JP2.17
PJ7  (via drill 0.5)
  Top 0.254: IC1.79 29.43,33.35 v30.32,33.35
  Bottom 0.254: v30.32,33.35 30.16,39.07 30.96,39.86 30.96,42.87 30.64,43.19 JP2.27
PK0
  Top 0.254: IC1.89 20.13,35.57 18.89,35.57 18.26,36.21 18.26,42.87 17.94,43.19 JP2.37
PK1
  Top 0.254: IC1.88 20.2,36.21 20,36.21 19.55,36.66 JP2.36
PK2
  Top 0.254: IC1.87 20.8,36.32 20.8,42.87 20.48,43.19 JP2.35
PK3
  Top 0.254: IC1.86 22.25,35.57 22.23,35.57 22.09,35.71 JP2.34
PK4
  Top 0.254: IC1.85 22.7,35.83 22.7,39.22 23.34,39.86 23.34,42.87 23.02,43.19 JP2.33
PK5
  Top 0.254: IC1.84 23.18,36.06 23.18,38.75 23.81,39.38 23.81,39.83 JP2.32
PK6
  Top 0.254: IC1.83 23.81,36.14 23.81,38.43 24.45,39.07 25.56,39.07 25.88,39.38 25.88,42.87 25.56,43.19 JP2.31
PK7
  Top 0.254: IC1.82 24.45,36.21 24.45,38.11 24.77,38.43 26.67,38.43 27.17,38.93 JP2.30
PL0  (via drill 0.5)
  Top 0.254: IC1.35 34.59,19.7 v33.34,19.7
  Bottom 0.254: JP1.32 39.84,6.2 41.27,7.63 42.86,7.63 43.81,8.58 43.81,14.62 38.73,19.7 v33.34,19.7
PL1  (via drill 0.5)
  Top 0.254: IC1.36 34.35,20.65 v32.7,20.65
  Bottom 0.254: JP1.33 41.48,2.5 41.12,2.87 41.12,6.36 41.75,7 43.18,7 44.45,8.27 44.45,14.93 38.73,20.65 v32.7,20.65
PL2  (via drill 0.5)
  Top 0.254: IC1.37 34.1,21.6 v33.34,21.6
  Bottom 0.254: JP1.34 42.38,6.2 42.55,6.36 43.5,6.36 45.09,7.95 45.09,15.25 39.05,21.29 34.29,21.29 33.97,21.6 v33.34,21.6
PL3  (via drill 0.5)
  Top 0.254: IC1.38 34.29,22.12 v34.29,22.56
  Bottom 0.254: JP1.35 44.02,2.5 43.66,2.87 43.66,5.57 45.72,7.63 45.72,15.57 39.37,21.92 34.92,21.92 v34.29,22.56
PL4  (via drill 0.5)
  Top 0.254: IC1.39 35.56,21.56 v35.56,23.19
  Bottom 0.254: JP1.36 44.92,5.88 46.35,7.32 46.35,15.89 39.69,22.56 36.2,22.56 v35.56,23.19
PL5  (via drill 0.5)
  Top 0.254: IC1.40 36.2,21.63 36.2,22.56 v37.15,23.51
  Bottom 0.254: JP1.37 46.56,2.5 46.2,2.87 46.2,6.2 46.99,7 46.99,16.2 40.01,23.19 37.47,23.19 v37.15,23.51
PL6  (via drill 0.5)
  Top 0.254: IC1.41 37.15,21.39 37.15,22.24 v39.05,24.14
  Bottom 0.254: JP1.38 47.47,16.68 40.01,24.14 v39.05,24.14
PL7
  Top 0.254: IC1.42 38.33,20.93 44.13,15.13 44.13,10.17 48.9,5.41 48.9,3.19 49.58,2.5 JP1.39
RESET  (via drill 0.5)
  Top 0.254: 33.52,8.09 33.66,7.95 33.66,7 33.97,6.68 35.72,6.68 36.04,6.36 36.04,2.87 36.4,2.5 JP1.29 38.21,2.5 38.58,2.87 38.58,6.52 37.78,7.32 37.78,7.95 37.77,7.96 C9.1 | 33.52,8.09 R1.1 | 33.52,8.09 D1.A 31.11,7.96 v31.11,6.68 | IC1.30 35.19,15.57 v35.4,15.57
  Bottom 0.254: ISP.5 12.14,18.35 12.38,18.11 12.38,12.4 14.61,10.17 14.61,8.58 14.92,8.27 26.99,8.27 28.57,6.68 v31.11,6.68 31.11,17.47 31.43,17.79 33.18,17.79 v35.4,15.57
RXD0  (via drill 0.5)
  Top 0.254: v48.26,19.38 47.31,19.38 41.27,25.41 40.32,25.41 39.69,26.05 33.97,26.05 32.38,24.46 22.75,24.46 IC1.2 21.02,22.72 20.5,22.72 15.24,17.47 15.24,13.35 13.34,11.44 2.54,11.44 1.75,10.65 JP1.2 | IC3.9 56.88,18.15 v56.83,18.11
  Bottom 0.254: v48.26,19.38 55.56,19.38 v56.83,18.11
RXD1
  Top 0.254: IC1.45 46.04,15.33 46.04,11.13 49.53,7.63 52.07,7.63 52.55,7.16 JP1.42
RXD3  (via drill 0.5)
  Top 0.254: IC1.63 36.24,30.18 v34.29,30.18 | IC2.26 49.18,23.16 v48.9,22.87
  Bottom 0.254: v34.29,30.18 36.2,30.18 36.83,29.54 36.83,26.21 37.47,25.57 40.8,25.57 43.5,22.87 v48.9,22.87
T1OUT
  Top 0.305: IC3.13 54.28,16.86 54.75,16.38 RS232.1
TXD0  (via drill 0.5)
  Top 0.254: v48.26,18.11 47.62,18.11 40.96,24.78 40.01,24.78 39.37,25.41 34.29,25.41 32.7,23.82 22.82,23.82 IC1.3 21.26,22.24 20.88,22.24 15.86,17.2 15.88,13.03 13.65,10.81 3.65,10.81 3.02,10.17 3.02,2.87 3.38,2.5 JP1.3 | IC3.11 55.58,18.12 v55.56,18.11
  Bottom 0.254: v48.26,18.11 v55.56,18.11
TXD1
  Top 0.254: IC1.46 46.67,15.4 46.67,11.44 49.85,8.27 53.66,8.27 53.98,7.95 53.98,3.51 54.98,2.5 JP1.43
TXD3  (via drill 0.5)
  Top 0.254: IC1.64 37.44,32.08 v37.78,32.08 | IC2.25 48.68,23.93 48.26,23.51 46.99,23.51 46.67,23.82 v46.04,23.82
  Bottom 0.254: v37.78,32.08 37.47,31.76 37.47,26.52 37.78,26.21 41.12,26.21 43.5,23.82 v46.04,23.82
VBUS  (via drill 0.5)
  Top 0.254: IC2.8 50.62,29.04 50.8,29.22 51.12,29.22 | IC2.7 50.98,28.45 51.12,28.59 51.12,29.22 | USB.VBUS 56.73,25.83 57.15,25.41 v58.74,25.41 59.05,25.73 59.05,30.18 58.74,30.49 54.93,30.49 54.77,30.34 | 54.77,30.34 54.61,30.18 54.61,29.54 54.29,29.22 51.12,29.22 | 54.77,30.34 C16.1
  Bottom 0.254: SJ1.1 58.41,22.56 58.42,22.56 58.74,22.87 v58.74,25.41
VCC  (via drill 0.5)
  Top 0.254: IC1.31 34.41,17.04 33.34,18.11 31.43,18.11 31.15,18.14 | C3.2 39.69,32.76 39.69,32.21 IC1.61 | C4.2 26.99,35.02 26.99,34.94 27.13,34.94 IC1.80 | v51.75,32.4 52.07,32.08 52.07,30.81 52.39,31.13 56.52,31.13 56.83,31.45 56.83,32.72 56.85,32.7 R2.1 | C1.2 22.49,18.43 22.54,18.43 22.54,18.6 IC1.10
  Top 0.305: IC3.15 52.98,20.06 52.7,20.33 52.7,20.97 52.3,21.37 C10.2 | IC1.61 35.75,28.27 33.02,28.27 33.02,28.9 32.85,28.9 | 32.14,29.93 IC1.80 | 26.99,34.94 C4.2 | 20,24.46 20.32,24.78 22.23,24.78 22.86,25.41 24.13,25.41 | IC1.10 26.18,22.24 v26.99,22.24
  Top 0.406: C4.2 26.96,35.22 26.99,35.25 26.99,37.16 | 30.96,44.46 30.96,41.76 29.84,40.65 JP2.28 | R3.2 52.08,30.8 52.07,30.81 | 35.36,9.42 R1.2 35.42,8.09 35.56,7.95 36.2,7.95 36.51,7.63 36.51,7 37.3,6.21 JP1.30 | 35.36,9.42 35.24,9.54 31.75,9.54 31.31,9.98 D1.C | C2.1 36.76,10.42 36.51,10.17 36.51,9.85 36.2,9.54 35.56,9.54 35.45,9.42 35.36,9.42 | C17.+ 12.38,14.75 12.38,14.62 9.53,14.62 8.18,13.27 ISP.2 | v43.81,26.05 43.81,24.78 47.62,20.97 51.12,20.97 51.44,21.29 52.07,21.29 52.16,21.37 C10.2 52.23,21.45 52.07,21.6 v52.07,22.56 | 32.14,29.93 v33.81,31.6
  Top 0.61: 32.14,29.93 32.85,29.22 32.85,28.9 32.85,26.19 32.07,25.41 v26.99,25.41 24.13,25.41 | JP2.28 29.71,39.25 28.89,38.43 28.26,38.43 26.99,37.16 | JP2.48 4.76,40.2 4.76,36.53 4.68,36.53 JP3.3 2.83,36.5 2.22,35.89 2.22,27.63 3.21,26.65 5.71,26.65 | ISP.2 6.74,13.27 5.71,14.3 5.71,26.65 | JP2.11 50.03,43.96 49.21,44.78 31.27,44.78 30.96,44.46 | C17.+ 13.42,19.46 13.97,20.02 15.56,20.02 20,24.46 | v26.99,22.24 31.11,18.11 31.18,18.11 31.15,18.14 31.15,11.47 | 31.15,11.47 31.16,11.49 D1.C | 31.15,11.47 31.11,11.44 | 5.71,26.65 8.86,26.65 9.21,27 10.79,27 10.83,26.97 L1.1
  Bottom 0.254: SJ1.2 55.87,23.2 54.93,24.14 54.93,26.36 54.61,26.68 51.12,26.68
  Bottom 0.406: v52.07,22.56 51.75,22.56 51.12,23.19 51.12,26.68 51.12,31.76 v51.75,32.4 | v43.81,26.05 43.81,27.32 43.18,27.95 40.01,27.95 39.05,28.9 39.05,32.08 38.1,33.03 35.24,33.03 v33.81,31.6
  Bottom 0.61: v26.99,25.41 v26.99,22.24
  Bottom 0.813: JP1.10 11.9,7.79 11.43,8.27 8.89,8.27 7.99,9.17 ISP.2
XTAL1
  Top 0.254: 39.04,12.71 39.05,12.71 | 39.04,12.71 Q2.3 | 39.04,12.71 C7.1 36.51,12.71 36.2,13.03 36.2,15.09 36.35,15.25 36.35,16.52 36.2,16.68 | IC1.33 36.2,16.68 | 36.2,16.68
XTAL2
  Top 0.254: IC1.34 36.74,16.84 39.69,16.84 41.28,15.25 Q2.1 41.27,14.3 43.13,14.3 C8.1

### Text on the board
Top: BS
Bottom: RN-Mega2560 Modul | robotikhardware.de | LS
tPlace: Pin1 | Pin50 | TX | V 1.3 | RN-Mega2560 Modul | RX | Pin50 | Pin1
